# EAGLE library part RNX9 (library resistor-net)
RESISTOR NETWORK
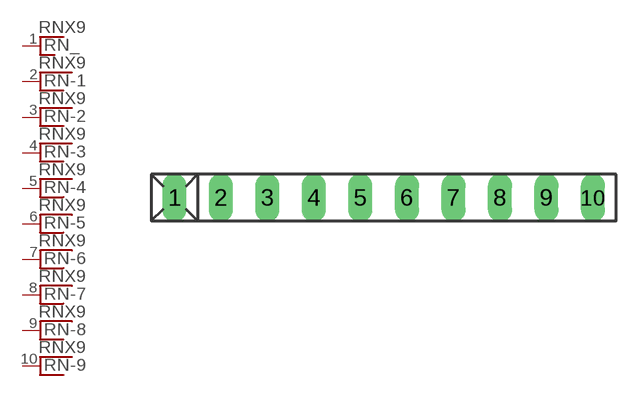
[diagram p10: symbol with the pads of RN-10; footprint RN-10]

Designator prefix RN; gates _=RN_1 -1=RNX -2=RNX -3=RNX -4=RNX -5=RNX -6=RNX -7=RNX -8=RNX -9=RNX

## RNX9 (OC_FARNELL: unknown; OC_NEWARK: unknown)  [RN-10]
1  _:1  pas
2  -1:1  pas
3  -2:1  pas
4  -3:1  pas
5  -4:1  pas
6  -5:1  pas
7  -6:1  pas
8  -7:1  pas
9  -8:1  pas
10  -9:1  pas

## Footprint RN-10 (pad centres in mm)
RESISTOR NETWORK
drill 0.813 long: 1 -11.43,0; 2 -8.89,0; 3 -6.35,0; 4 -3.81,0; 5 -1.27,0; 6 1.27,0; 7 3.81,0; 8 6.35,0; 9 8.89,0; 10 11.43,0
